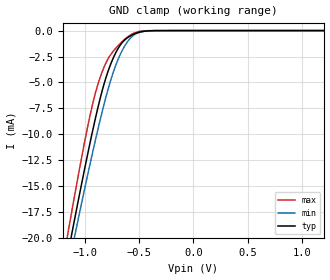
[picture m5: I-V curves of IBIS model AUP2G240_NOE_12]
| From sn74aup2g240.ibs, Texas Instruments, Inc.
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[Model]   AUP2G240_NOE_12
Model_type  Input
Vinl=0.420
Vinh=0.715
| variable   typ   min   max
C_comp   1.50pF   1.33pF   1.79pF
[Temperature Range]   40   100   -40
| Ambient temperature   25   85   -40
[Voltage range]   1.2   1.1   1.3
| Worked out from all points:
|   GND clamp passes 1 mA (typ) near -0.64 V on its own axis
[GND Clamp]
| AUP2G240_NOE_12
|   Voltage   I(typ)   I(min)   I(max)
-3.6V     -169.6mA   -161.4mA   -179.1mA
-1.165V   -22.22mA   -23.63mA   -20.26mA
-1.14V    -20.84mA   -22.34mA   -18.78mA
-1.115V   -19.48mA   -21.06mA   -17.3mA
-1.095V   -18.4mA    -20.04mA   -16.13mA
-1.075V   -17.32mA   -19.03mA   -14.97mA
-950mV    -10.86mA   -12.9mA    -8.222mA
-850mV    -6.292mA   -8.346mA   -4.331mA
-710mV    -2.081mA   -3.263mA   -1.67mA
-560mV    -408.5uA   -545.4uA   -322.3uA
-345mV    -4.449uA   -6.656uA   -797.7nA
1.2V      66.98pA    416.9pA    12.63pA
